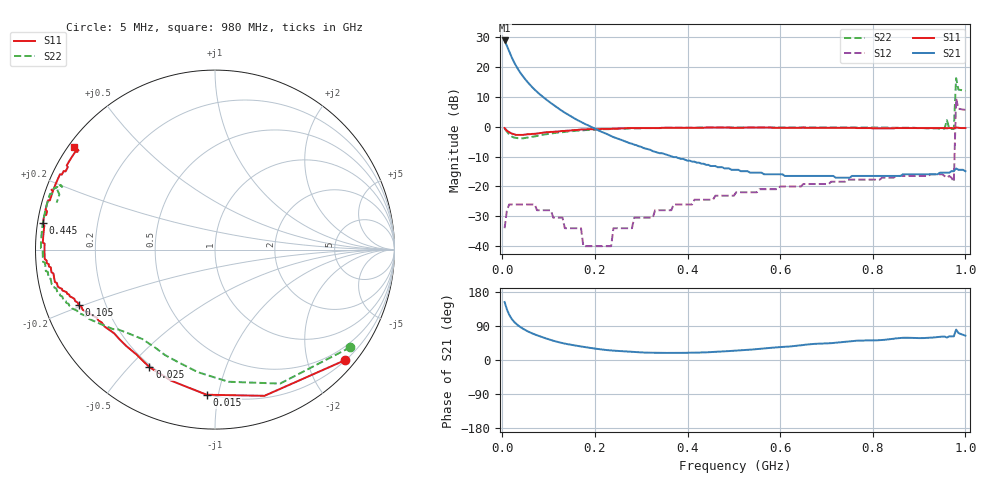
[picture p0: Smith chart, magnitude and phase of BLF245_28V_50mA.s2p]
! Filename:  BLF245_28V_50mA.s2p
! Philips part #: BLF245  !date: 22-05-2003
!Vdd=28V ; Idq=50 mA
!D:\Vee measurements\measurement data\VDMOST\BLF245\28V_50mA_#1
# HZ S MA R 50
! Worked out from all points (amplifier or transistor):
!   200 points, 5 MHz to 1 GHz, reference 50 ohm
!   highest |S21| = 28.9 dB at 5 MHz (marker M1)
!   |S21| within 3 dB of that: start of sweep to 13.15 MHz
!   unconditionally stable (mu >= 1): 174.3 MHz to 188.7 MHz; 190.8 MHz to 236.4 MHz; 654.9 MHz to 955.6 MHz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
!   at 170 MHz: K = 0.20, MSG = 17.8 dB, |S12| = -34.0 dB
!   at 505 MHz: K = 0.73, MSG = 3.8 dB, |S12| = -21.9 dB
!   at 1 GHz: K = -2.30, MSG = -10.3 dB, |S12| = 5.7 dB
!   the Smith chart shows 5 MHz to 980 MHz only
!   S11 on the Smith chart (normalised r, x): 5 MHz: 0.21, -2.70; 15 MHz: 0.20, -0.92; 25 MHz: 0.19, -0.57; 105 MHz: 0.10, -0.19; 445 MHz: 0.02, +0.08; 980 MHz: 0.02, +0.33
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5000000  0.95 -40.5  27.84 152.9  0.02 63.8  0.93 -35.8
1e7  0.86 -71.3  22.6 133.3  0.04 44.4  0.83 -64.1
1.5e7  0.81 -93.3  18.19 119.2  0.05 30.8  0.74 -84.2
2e7  0.77 -108.6  14.77 109.1  0.05 21.7  0.69 -97.8
2.5e7  0.75 -119.2  12.24 101.4  0.05 14.6  0.66 -108.1
3.5e7  0.73 -132.4  8.93 90.5  0.05 4.7  0.64 -121.0
5.5e7  0.75 -145.2  5.54 75.6  0.05 -7.4  0.66 -133.6
7.5e7  0.77 -151.2  3.84 65.2  0.04 -14.8  0.7 -140.6
1.05e8  0.82 -157.8  2.49 52.8  0.04 -21.8  0.77 -148.1
1.75e8  0.9 -167.4  1.15 34.7  0.01 -5.0  0.87 -159.7
3.4e8  0.95 178.0  0.36 18.9  0.04 87.2  0.95 -175.3
4.45e8  0.97 171.3  0.23 20.5  0.06 87.5  0.97 178.4
5.05e8  0.96 167.9  0.19 24.6  0.08 85.9  0.97 175.2
6.7e8  0.96 158.9  0.15 42.2  0.11 82.5  0.97 167.8
8.35e8  0.94 151.1  0.15 54.5  0.14 80.8  0.96 161.1
9.5e8  0.95 145.2  0.17 61.7  0.16 74.9  0.93 157.3
9.6e8  0.94 144.6  0.17 59.3  0.14 -144.0  1.29 -172.3
9.65e8  0.95 144.4  0.17 62.4  0.15 75.6  0.94 159.2
9.75e8  0.94 144.0  0.18 62.5  0.12 69.9  0.92 163.5
9.8e8  0.97 143.9  0.2 80.2  2.96 61.5  6.5 64.5
9.85e8  0.96 143.5  0.19 71.3  2 55.8  4.19 62.3
1e9  0.95 142.9  0.18 64.3  1.92 53.7  4.01 59.9
